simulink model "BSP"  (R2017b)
settings: Solver=FixedStepDiscrete  StartTime=0.0  StopTime=10.0  FixedStep=0.01  RelTol=1e-3  EnableMultiTasking=on
undefined symbols (not defined in the file): ASWTYPE_FALSE, ASWTYPE_TRUE, CcBSP_CellVoltRngHiThrd_mV, CcBSP_CellVoltRngLowThrd_mV, CcBSP_ChrgMaxCellTempSaf_C, CcBSP_DCChrgNegTempHiThrd_C, CcBSP_DCChrgPosTempHiThrd_C, CcBSP_MaxCellTempSaf_C, CcBSP_MaxCellVoltSafDiff_mV, CcBSP_MinCellVoltSafDiff_mV, CcBSP_PackCurrSaf_A, Enum_CTCCtrCtlConnMode, Enum_LDPCC2St, Enum_ODPCCState
libraries: AIWAYS_Powertrain_BMS_lib x14

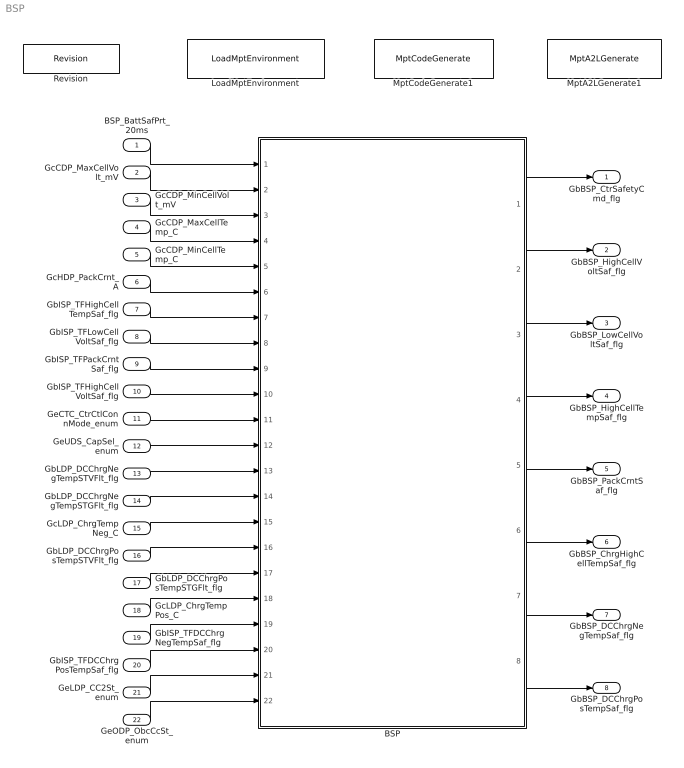
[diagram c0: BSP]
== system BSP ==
  BSP_BattSafPrt_20ms : Inport
  GcCDP_MaxCellVolt_mV : Inport  Port=2
  GcCDP_MinCellVolt_mV : Inport  Port=3
  GcCDP_MaxCellTemp_C : Inport  Port=4
  GcCDP_MinCellTemp_C : Inport  Port=5
  GcHDP_PackCrnt_A : Inport  Port=6
  GbISP_TFHighCellTempSaf_flg : Inport  Port=7
  GbISP_TFLowCellVoltSaf_flg : Inport  Port=8
  GbISP_TFPackCrntSaf_flg : Inport  Port=9
  GbISP_TFHighCellVoltSaf_flg : Inport  Port=10
  GeCTC_CtrCtlConnMode_enum : Inport  Port=11
  GeUDS_CapSel_enum : Inport  Port=12
  GbLDP_DCChrgNegTempSTVFlt_flg : Inport  Port=13
  GbLDP_DCChrgNegTempSTGFlt_flg : Inport  Port=14
  GcLDP_ChrgTempNeg_C : Inport  Port=15
  GbLDP_DCChrgPosTempSTVFlt_flg : Inport  Port=16
  GbLDP_DCChrgPosTempSTGFlt_flg : Inport  Port=17
  GcLDP_ChrgTempPos_C : Inport  Port=18
  GbISP_TFDCChrgNegTempSaf_flg : Inport  Port=19
  GbISP_TFDCChrgPosTempSaf_flg : Inport  Port=20
  GeLDP_CC2St_enum : Inport  Port=21
  GeODP_ObcCcSt_enum : Inport  Port=22
  BSP : Subsystem
  LoadMptEnvironment : AIWAYS_Powertrain_BMS_lib/Config/LoadMptEnvironment  ProjectName=Comm  SuppierID=NewPlatformUAES
  MptA2LGenerate1 : AIWAYS_Powertrain_BMS_lib/Config/MptA2LGenerate  SystemSampleTime=-1
  MptCodeGenerate1 : AIWAYS_Powertrain_BMS_lib/Config/MptCodeGenerate  SystemSampleTime=-1
  Revision : AIWAYS_Powertrain_BMS_lib/Config/Revision  curVersion='M105C111'  newVersion='M105C111'
  GbBSP_CtrSafetyCmd_flg : Outport
  GbBSP_HighCellVoltSaf_flg : Outport  Port=2
  GbBSP_LowCellVoltSaf_flg : Outport  Port=3
  GbBSP_HighCellTempSaf_flg : Outport  Port=4
  GbBSP_PackCrntSaf_flg : Outport  Port=5
  GbBSP_ChrgHighCellTempSaf_flg : Outport  Port=6
  GbBSP_DCChrgNegTempSaf_flg : Outport  Port=7
  GbBSP_DCChrgPosTempSaf_flg : Outport  Port=8
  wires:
  GcCDP_MaxCellVolt_mV/1 -> BSP/2(GcCDP_MaxCellVolt_mV)
  GcCDP_MinCellVolt_mV/1 -> BSP/3(GcCDP_MinCellVolt_mV)
  GcCDP_MaxCellTemp_C/1 -> BSP/4(GcCDP_MaxCellTemp_C)
  GcCDP_MinCellTemp_C/1 -> BSP/5(GcCDP_MinCellTemp_C)
  GcHDP_PackCrnt_A/1 -> BSP/6(GcHDP_PackCrnt_A)
  BSP_BattSafPrt_20ms/1 -> BSP/1(BSP_BattSafPrt_20ms)
  BSP/1(GbBSP_CtrSafetyCmd_flg) -> GbBSP_CtrSafetyCmd_flg/1
  BSP/2(GbBSP_HighCellVoltSaf_flg) -> GbBSP_HighCellVoltSaf_flg/1
  BSP/3(GbBSP_LowCellVoltSaf_flg) -> GbBSP_LowCellVoltSaf_flg/1
  BSP/4(GbBSP_HighCellTempSaf_flg) -> GbBSP_HighCellTempSaf_flg/1
  BSP/5(GbBSP_PackCrntSaf_flg) -> GbBSP_PackCrntSaf_flg/1
  GbISP_TFHighCellTempSaf_flg/1 -> BSP/7(GbISP_TFHighCellTempSaf_flg)
  GbISP_TFLowCellVoltSaf_flg/1 -> BSP/8(GbISP_TFLowCellVoltSaf_flg)
  GbISP_TFPackCrntSaf_flg/1 -> BSP/9(GbISP_TFPackCrntSaf_flg)
  GbISP_TFHighCellVoltSaf_flg/1 -> BSP/10(GbISP_TFHighCellVoltSaf_flg)
  BSP/6(GbBSP_ChrgHighCellTempSaf_flg) -> GbBSP_ChrgHighCellTempSaf_flg/1
  GeCTC_CtrCtlConnMode_enum/1 -> BSP/11(GeCTC_CtrCtlConnMode_enum)
  GeUDS_CapSel_enum/1 -> BSP/12(GeUDS_CapSel_enum)
  GbLDP_DCChrgNegTempSTVFlt_flg/1 -> BSP/13(GbLDP_DCChrgNegTempSTVFlt_flg)
  GbLDP_DCChrgNegTempSTGFlt_flg/1 -> BSP/14(GbLDP_DCChrgNegTempSTGFlt_flg)
  GcLDP_ChrgTempNeg_C/1 -> BSP/15(GcLDP_ChrgTempNeg_C)
  GbLDP_DCChrgPosTempSTVFlt_flg/1 -> BSP/16(GbLDP_DCChrgPosTempSTVFlt_flg)
  GbLDP_DCChrgPosTempSTGFlt_flg/1 -> BSP/17(GbLDP_DCChrgPosTempSTGFlt_flg)
  GcLDP_ChrgTempPos_C/1 -> BSP/18(GcLDP_ChrgTempPos_C)
  GbISP_TFDCChrgNegTempSaf_flg/1 -> BSP/19(GbISP_TFDCChrgNegTempSaf_flg)
  GbISP_TFDCChrgPosTempSaf_flg/1 -> BSP/20(GbISP_TFDCChrgPosTempSaf_flg)
  BSP/7(GbBSP_DCChrgNegTempSaf_flg) -> GbBSP_DCChrgNegTempSaf_flg/1
  BSP/8(GbBSP_DCChrgPosTempSaf_flg) -> GbBSP_DCChrgPosTempSaf_flg/1
  GeLDP_CC2St_enum/1 -> BSP/21(GeLDP_CC2St_enum)
  GeODP_ObcCcSt_enum/1 -> BSP/22(GeODP_ObcCcSt_enum)

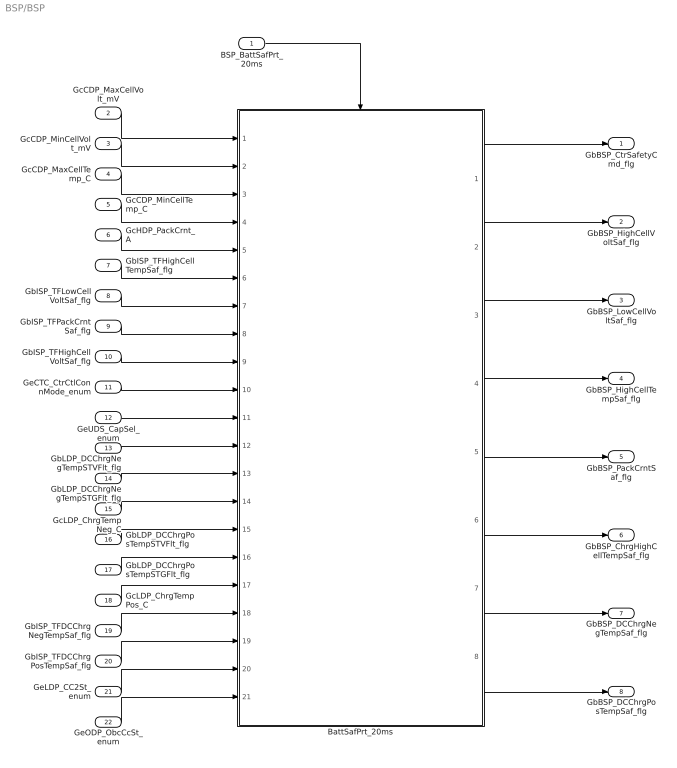
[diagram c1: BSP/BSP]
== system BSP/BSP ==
  BSP_BattSafPrt_20ms : Inport
  GcCDP_MaxCellVolt_mV : Inport  Port=2
  GcCDP_MinCellVolt_mV : Inport  Port=3
  GcCDP_MaxCellTemp_C : Inport  Port=4
  GcCDP_MinCellTemp_C : Inport  Port=5
  GcHDP_PackCrnt_A : Inport  Port=6
  GbISP_TFHighCellTempSaf_flg : Inport  Port=7
  GbISP_TFLowCellVoltSaf_flg : Inport  Port=8
  GbISP_TFPackCrntSaf_flg : Inport  Port=9
  GbISP_TFHighCellVoltSaf_flg : Inport  Port=10
  GeCTC_CtrCtlConnMode_enum : Inport  Port=11
  GeUDS_CapSel_enum : Inport  Port=12
  GbLDP_DCChrgNegTempSTVFlt_flg : Inport  Port=13
  GbLDP_DCChrgNegTempSTGFlt_flg : Inport  Port=14
  GcLDP_ChrgTempNeg_C : Inport  Port=15
  GbLDP_DCChrgPosTempSTVFlt_flg : Inport  Port=16
  GbLDP_DCChrgPosTempSTGFlt_flg : Inport  Port=17
  GcLDP_ChrgTempPos_C : Inport  Port=18
  GbISP_TFDCChrgNegTempSaf_flg : Inport  Port=19
  GbISP_TFDCChrgPosTempSaf_flg : Inport  Port=20
  GeLDP_CC2St_enum : Inport  Port=21
  GeODP_ObcCcSt_enum : Inport  Port=22
  BattSafPrt_20ms : Subsystem
  GbBSP_CtrSafetyCmd_flg : Outport
  GbBSP_HighCellVoltSaf_flg : Outport  Port=2
  GbBSP_LowCellVoltSaf_flg : Outport  Port=3
  GbBSP_HighCellTempSaf_flg : Outport  Port=4
  GbBSP_PackCrntSaf_flg : Outport  Port=5
  GbBSP_ChrgHighCellTempSaf_flg : Outport  Port=6
  GbBSP_DCChrgNegTempSaf_flg : Outport  Port=7
  GbBSP_DCChrgPosTempSaf_flg : Outport  Port=8
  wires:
  BSP_BattSafPrt_20ms/1 -> BattSafPrt_20ms/Trigger
  GcCDP_MaxCellVolt_mV/1 -> BattSafPrt_20ms/1(GcCDP_MaxCellVolt_mV)
  GcCDP_MinCellVolt_mV/1 -> BattSafPrt_20ms/2(GcCDP_MinCellVolt_mV)
  GcCDP_MaxCellTemp_C/1 -> BattSafPrt_20ms/3(GcCDP_MaxCellTemp_C)
  GcCDP_MinCellTemp_C/1 -> BattSafPrt_20ms/4(GcCDP_MinCellTemp_C)
  GcHDP_PackCrnt_A/1 -> BattSafPrt_20ms/5(GcHDP_PackCrnt_A)
  BattSafPrt_20ms/1(GbBSP_CtrSafetyCmd_flg) -> GbBSP_CtrSafetyCmd_flg/1
  BattSafPrt_20ms/2(GbBSP_HighCellVoltSaf_flg) -> GbBSP_HighCellVoltSaf_flg/1
  BattSafPrt_20ms/3(GbBSP_LowCellVoltSaf_flg) -> GbBSP_LowCellVoltSaf_flg/1
  BattSafPrt_20ms/4(GbBSP_HighCellTempSaf_flg) -> GbBSP_HighCellTempSaf_flg/1
  BattSafPrt_20ms/5(GbBSP_PackCrntSaf_flg) -> GbBSP_PackCrntSaf_flg/1
  GbISP_TFHighCellTempSaf_flg/1 -> BattSafPrt_20ms/6(GbISP_TFHighCellTempSaf_flg)
  GbISP_TFLowCellVoltSaf_flg/1 -> BattSafPrt_20ms/7(GbISP_TFLowCellVoltSaf_flg)
  GbISP_TFPackCrntSaf_flg/1 -> BattSafPrt_20ms/8(GbISP_TFPackCrntSaf_flg)
  GbISP_TFHighCellVoltSaf_flg/1 -> BattSafPrt_20ms/9(GbISP_TFHighCellVoltSaf_flg)
  GeCTC_CtrCtlConnMode_enum/1 -> BattSafPrt_20ms/10(GeCTC_CtrCtlConnMode_enum)
  BattSafPrt_20ms/6(GbBSP_ChrgHighCellTempSaf_flg) -> GbBSP_ChrgHighCellTempSaf_flg/1
  GeUDS_CapSel_enum/1 -> BattSafPrt_20ms/11(GeUDS_CapSel_enum)
  GbLDP_DCChrgNegTempSTVFlt_flg/1 -> BattSafPrt_20ms/12(GbLDP_DCChrgNegTempSTVFlt_flg)
  GbLDP_DCChrgNegTempSTGFlt_flg/1 -> BattSafPrt_20ms/13(GbLDP_DCChrgNegTempSTGFlt_flg)
  GcLDP_ChrgTempNeg_C/1 -> BattSafPrt_20ms/14(GcLDP_ChrgTempNeg_C)
  GbLDP_DCChrgPosTempSTVFlt_flg/1 -> BattSafPrt_20ms/15(GbLDP_DCChrgPosTempSTVFlt_flg)
  GbLDP_DCChrgPosTempSTGFlt_flg/1 -> BattSafPrt_20ms/16(GbLDP_DCChrgPosTempSTGFlt_flg)
  GcLDP_ChrgTempPos_C/1 -> BattSafPrt_20ms/17(GcLDP_ChrgTempPos_C)
  GbISP_TFDCChrgNegTempSaf_flg/1 -> BattSafPrt_20ms/18(GbISP_TFDCChrgNegTempSaf_flg)
  GbISP_TFDCChrgPosTempSaf_flg/1 -> BattSafPrt_20ms/19(GbISP_TFDCChrgPosTempSaf_flg)
  BattSafPrt_20ms/7(GbBSP_DCChrgNegTempSaf_flg) -> GbBSP_DCChrgNegTempSaf_flg/1
  BattSafPrt_20ms/8(GbBSP_DCChrgPosTempSaf_flg) -> GbBSP_DCChrgPosTempSaf_flg/1
  GeLDP_CC2St_enum/1 -> BattSafPrt_20ms/20(GeLDP_CC2St_enum)
  GeODP_ObcCcSt_enum/1 -> BattSafPrt_20ms/21(GeODP_ObcCcSt_enum)

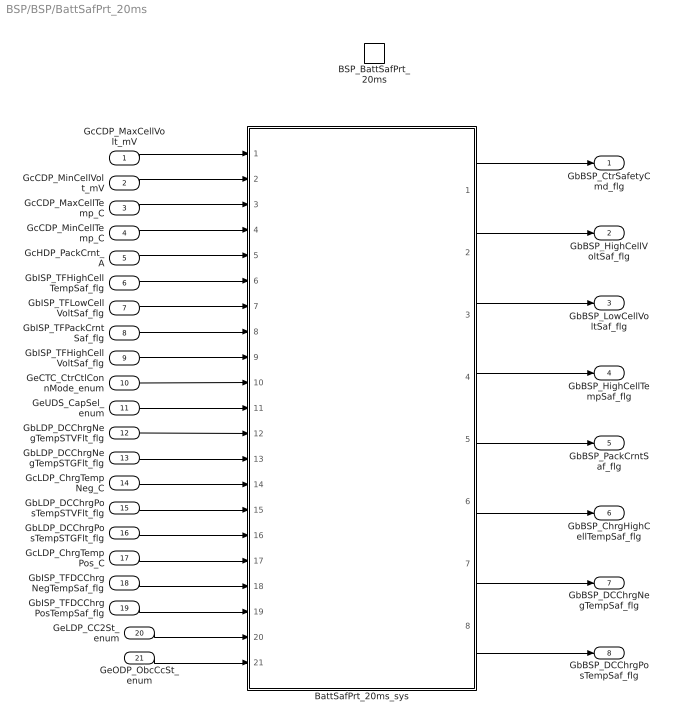
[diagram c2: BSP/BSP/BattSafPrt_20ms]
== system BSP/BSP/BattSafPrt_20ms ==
  GcCDP_MaxCellVolt_mV : Inport
  GcCDP_MinCellVolt_mV : Inport  Port=2
  GcCDP_MaxCellTemp_C : Inport  Port=3
  GcCDP_MinCellTemp_C : Inport  Port=4
  GcHDP_PackCrnt_A : Inport  Port=5
  GbISP_TFHighCellTempSaf_flg : Inport  Port=6
  GbISP_TFLowCellVoltSaf_flg : Inport  Port=7
  GbISP_TFPackCrntSaf_flg : Inport  Port=8
  GbISP_TFHighCellVoltSaf_flg : Inport  Port=9
  GeCTC_CtrCtlConnMode_enum : Inport  Port=10
  GeUDS_CapSel_enum : Inport  Port=11
  GbLDP_DCChrgNegTempSTVFlt_flg : Inport  Port=12
  GbLDP_DCChrgNegTempSTGFlt_flg : Inport  Port=13
  GcLDP_ChrgTempNeg_C : Inport  Port=14
  GbLDP_DCChrgPosTempSTVFlt_flg : Inport  Port=15
  GbLDP_DCChrgPosTempSTGFlt_flg : Inport  Port=16
  GcLDP_ChrgTempPos_C : Inport  Port=17
  GbISP_TFDCChrgNegTempSaf_flg : Inport  Port=18
  GbISP_TFDCChrgPosTempSaf_flg : Inport  Port=19
  GeLDP_CC2St_enum : Inport  Port=20
  GeODP_ObcCcSt_enum : Inport  Port=21
  BSP_BattSafPrt_20ms : TriggerPort  TriggerType=function-call  VariantControl=(inherit)
  BattSafPrt_20ms_sys : Subsystem
  GbBSP_CtrSafetyCmd_flg : Outport
  GbBSP_HighCellVoltSaf_flg : Outport  Port=2
  GbBSP_LowCellVoltSaf_flg : Outport  Port=3
  GbBSP_HighCellTempSaf_flg : Outport  Port=4
  GbBSP_PackCrntSaf_flg : Outport  Port=5
  GbBSP_ChrgHighCellTempSaf_flg : Outport  Port=6
  GbBSP_DCChrgNegTempSaf_flg : Outport  Port=7
  GbBSP_DCChrgPosTempSaf_flg : Outport  Port=8
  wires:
  GcCDP_MaxCellVolt_mV/1 -> BattSafPrt_20ms_sys/1(GcCDP_MaxCellVolt_mV)
  GcCDP_MinCellVolt_mV/1 -> BattSafPrt_20ms_sys/2(GcCDP_MinCellVolt_mV)
  GcCDP_MaxCellTemp_C/1 -> BattSafPrt_20ms_sys/3(GcCDP_MaxCellTemp_C)
  GcCDP_MinCellTemp_C/1 -> BattSafPrt_20ms_sys/4(GcCDP_MinCellTemp_C)
  GcHDP_PackCrnt_A/1 -> BattSafPrt_20ms_sys/5(GcHDP_PackCrnt_A)
  BattSafPrt_20ms_sys/1(GbBSP_CtrSafetyCmd_flg) -> GbBSP_CtrSafetyCmd_flg/1
  BattSafPrt_20ms_sys/2(GbBSP_HighCellVoltSaf_flg) -> GbBSP_HighCellVoltSaf_flg/1
  BattSafPrt_20ms_sys/3(GbBSP_LowCellVoltSaf_flg) -> GbBSP_LowCellVoltSaf_flg/1
  BattSafPrt_20ms_sys/4(GbBSP_HighCellTempSaf_flg) -> GbBSP_HighCellTempSaf_flg/1
  BattSafPrt_20ms_sys/5(GbBSP_PackCrntSaf_flg) -> GbBSP_PackCrntSaf_flg/1
  GbISP_TFHighCellTempSaf_flg/1 -> BattSafPrt_20ms_sys/6(GbISP_TFHighCellTempSaf_flg)
  GbISP_TFLowCellVoltSaf_flg/1 -> BattSafPrt_20ms_sys/7(GbISP_TFLowCellVoltSaf_flg)
  GbISP_TFPackCrntSaf_flg/1 -> BattSafPrt_20ms_sys/8(GbISP_TFPackCrntSaf_flg)
  GbISP_TFHighCellVoltSaf_flg/1 -> BattSafPrt_20ms_sys/9(GbISP_TFHighCellVoltSaf_flg)
  BattSafPrt_20ms_sys/6(GbBSP_ChrgHighCellTempSaf_flg) -> GbBSP_ChrgHighCellTempSaf_flg/1
  GeCTC_CtrCtlConnMode_enum/1 -> BattSafPrt_20ms_sys/10(GeCTC_CtrCtlConnMode_enum)
  GeUDS_CapSel_enum/1 -> BattSafPrt_20ms_sys/11(GeUDS_CapSel_enum)
  GbLDP_DCChrgNegTempSTVFlt_flg/1 -> BattSafPrt_20ms_sys/12(GbLDP_DCChrgNegTempSTVFlt_flg)
  GbLDP_DCChrgNegTempSTGFlt_flg/1 -> BattSafPrt_20ms_sys/13(GbLDP_DCChrgNegTempSTGFlt_flg)
  GcLDP_ChrgTempNeg_C/1 -> BattSafPrt_20ms_sys/14(GcLDP_ChrgTempNeg_C)
  GbLDP_DCChrgPosTempSTVFlt_flg/1 -> BattSafPrt_20ms_sys/15(GbLDP_DCChrgPosTempSTVFlt_flg)
  GbLDP_DCChrgPosTempSTGFlt_flg/1 -> BattSafPrt_20ms_sys/16(GbLDP_DCChrgPosTempSTGFlt_flg)
  GcLDP_ChrgTempPos_C/1 -> BattSafPrt_20ms_sys/17(GcLDP_ChrgTempPos_C)
  GbISP_TFDCChrgNegTempSaf_flg/1 -> BattSafPrt_20ms_sys/18(GbISP_TFDCChrgNegTempSaf_flg)
  GbISP_TFDCChrgPosTempSaf_flg/1 -> BattSafPrt_20ms_sys/19(GbISP_TFDCChrgPosTempSaf_flg)
  BattSafPrt_20ms_sys/8(GbBSP_DCChrgPosTempSaf_flg) -> GbBSP_DCChrgPosTempSaf_flg/1
  BattSafPrt_20ms_sys/7(GbBSP_DCChrgNegTempSaf_flg) -> GbBSP_DCChrgNegTempSaf_flg/1
  GeLDP_CC2St_enum/1 -> BattSafPrt_20ms_sys/20(GeLDP_CC2St_enum)
  GeODP_ObcCcSt_enum/1 -> BattSafPrt_20ms_sys/21(GeODP_ObcCcSt_enum)

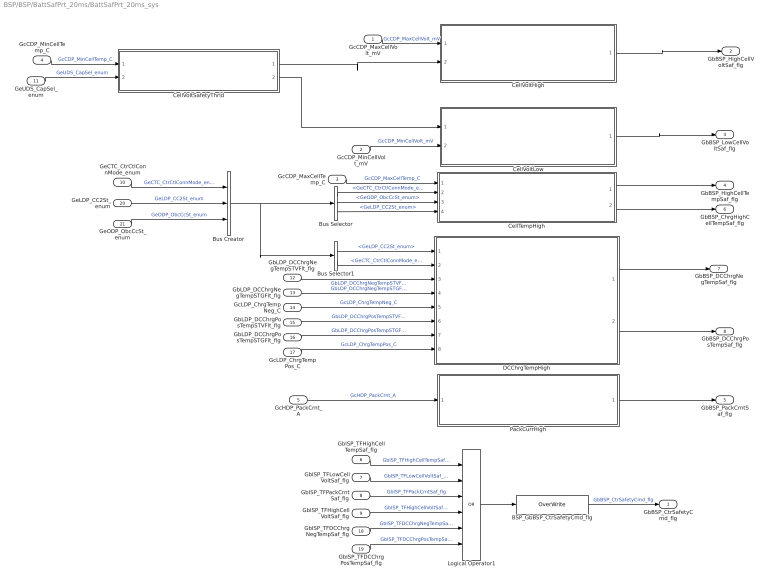
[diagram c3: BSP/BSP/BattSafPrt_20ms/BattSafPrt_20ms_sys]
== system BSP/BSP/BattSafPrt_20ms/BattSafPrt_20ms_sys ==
  GcCDP_MaxCellVolt_mV : Inport
  GcCDP_MinCellVolt_mV : Inport  Port=2
  GcCDP_MaxCellTemp_C : Inport  Port=3
  GcCDP_MinCellTemp_C : Inport  Port=4
  GcHDP_PackCrnt_A : Inport  Port=5
  GbISP_TFHighCellTempSaf_flg : Inport  Port=6
  GbISP_TFLowCellVoltSaf_flg : Inport  Port=7
  GbISP_TFPackCrntSaf_flg : Inport  Port=8
  GbISP_TFHighCellVoltSaf_flg : Inport  Port=9
  GeCTC_CtrCtlConnMode_enum : Inport  Port=10
  GeUDS_CapSel_enum : Inport  Port=11
  GbLDP_DCChrgNegTempSTVFlt_flg : Inport  Port=12
  GbLDP_DCChrgNegTempSTGFlt_flg : Inport  Port=13
  GcLDP_ChrgTempNeg_C : Inport  Port=14
  GbLDP_DCChrgPosTempSTVFlt_flg : Inport  Port=15
  GbLDP_DCChrgPosTempSTGFlt_flg : Inport  Port=16
  GcLDP_ChrgTempPos_C : Inport  Port=17
  GbISP_TFDCChrgNegTempSaf_flg : Inport  Port=18
  GbISP_TFDCChrgPosTempSaf_flg : Inport  Port=19
  GeLDP_CC2St_enum : Inport  Port=20
  GeODP_ObcCcSt_enum : Inport  Port=21
  BSP_GbBSP_CtrSafetyCmd_flg : AIWAYS_Powertrain_BMS_lib/Signals/OverWrite  OverWrite_Value=CbBSP_CtrSafetyCmdOvr_flg  OverWrite_flag=CbBSP_CtrSafetyCmdOvrSwt_flg
  Bus Creator : BusCreator  Inputs=3
  Bus Selector : BusSelector  OutputSignals=GeCTC_CtrCtlConnMode_enum,GeODP_ObcCcSt_enum,GeLDP_CC2St_enum
  Bus Selector1 : BusSelector  OutputSignals=GeLDP_CC2St_enum,GeCTC_CtrCtlConnMode_enum
  CellTempHigh : Subsystem
  CellVoltHigh : Subsystem
  CellVoltLow : Subsystem
  CellVoltSafetyThrld : Subsystem
  DCChrgTempHigh : Subsystem
  Logical Operator1 : Logic  Operator=OR  Inputs=6  AllPortsSameDT=off  OutDataTypeStr=boolean
  PackCurrHigh : Subsystem
  GbBSP_CtrSafetyCmd_flg : Outport
  GbBSP_HighCellVoltSaf_flg : Outport  Port=2
  GbBSP_LowCellVoltSaf_flg : Outport  Port=3
  GbBSP_HighCellTempSaf_flg : Outport  Port=4
  GbBSP_PackCrntSaf_flg : Outport  Port=5
  GbBSP_ChrgHighCellTempSaf_flg : Outport  Port=6
  GbBSP_DCChrgNegTempSaf_flg : Outport  Port=7
  GbBSP_DCChrgPosTempSaf_flg : Outport  Port=8
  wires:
  GcCDP_MinCellTemp_C/1 -> CellVoltSafetyThrld/1(GcCDP_MinCellTemp_C)  "GcCDP_MinCellTemp_C"
  GcCDP_MaxCellVolt_mV/1 -> CellVoltHigh/1(GcCDP_MaxCellVolt_mV)  "GcCDP_MaxCellVolt_mV"
  CellVoltSafetyThrld/1(LcBSP_MaxCellVoltSafetyThrld_mV) -> CellVoltHigh/2(LcBSP_MaxCellVoltSafetyThrld_mV)
  CellVoltSafetyThrld/2(LcBSP_MinCellVoltSafetyThrld_mV) -> CellVoltLow/1(LcBSP_MinCellVoltSafetyThrld_mV)
  GcCDP_MinCellVolt_mV/1 -> CellVoltLow/2(GcCDP_MinCellVolt_mV)  "GcCDP_MinCellVolt_mV"
  GcCDP_MaxCellTemp_C/1 -> CellTempHigh/1(GcCDP_MaxCellTemp_C)  "GcCDP_MaxCellTemp_C"
  GcHDP_PackCrnt_A/1 -> PackCurrHigh/1(GcHDP_PackCrnt_A)  "GcHDP_PackCrnt_A"
  CellVoltHigh/1(GbBSP_HighCellVoltSaf_flg) -> GbBSP_HighCellVoltSaf_flg/1
  CellVoltLow/1(GbBSP_LowCellVoltSaf_flg) -> GbBSP_LowCellVoltSaf_flg/1
  CellTempHigh/1(GbBSP_HighCellTempSaf_flg) -> GbBSP_HighCellTempSaf_flg/1
  PackCurrHigh/1(GbBSP_PackCrntSaf_flg) -> GbBSP_PackCrntSaf_flg/1
  Logical Operator1/1 -> BSP_GbBSP_CtrSafetyCmd_flg/1
  BSP_GbBSP_CtrSafetyCmd_flg/1 -> GbBSP_CtrSafetyCmd_flg/1  "GbBSP_CtrSafetyCmd_flg"
  GbISP_TFHighCellTempSaf_flg/1 -> Logical Operator1/1  "GbISP_TFHighCellTempSaf_flg"
  GbISP_TFLowCellVoltSaf_flg/1 -> Logical Operator1/2  "GbISP_TFLowCellVoltSaf_flg"
  GbISP_TFPackCrntSaf_flg/1 -> Logical Operator1/3  "GbISP_TFPackCrntSaf_flg"
  GbISP_TFHighCellVoltSaf_flg/1 -> Logical Operator1/4  "GbISP_TFHighCellVoltSaf_flg"
  CellTempHigh/2(GbBSP_ChrgHighCellTempSaf_flg) -> GbBSP_ChrgHighCellTempSaf_flg/1
  GeUDS_CapSel_enum/1 -> CellVoltSafetyThrld/2(GeUDS_CapSel_enum)  "GeUDS_CapSel_enum"
  GbLDP_DCChrgNegTempSTVFlt_flg/1 -> DCChrgTempHigh/3(GbLDP_DCChrgNegTempSTVFlt_flg)  "GbLDP_DCChrgNegTempSTVFlt_flg"
  GbLDP_DCChrgNegTempSTGFlt_flg/1 -> DCChrgTempHigh/4(GbLDP_DCChrgNegTempSTGFlt_flg)  "GbLDP_DCChrgNegTempSTGFlt_flg"
  GcLDP_ChrgTempNeg_C/1 -> DCChrgTempHigh/5(GcLDP_ChrgTempNeg_C)  "GcLDP_ChrgTempNeg_C"
  GbLDP_DCChrgPosTempSTVFlt_flg/1 -> DCChrgTempHigh/6(GbLDP_DCChrgPosTempSTVFlt_flg)  "GbLDP_DCChrgPosTempSTVFlt_flg"
  GbLDP_DCChrgPosTempSTGFlt_flg/1 -> DCChrgTempHigh/7(GbLDP_DCChrgPosTempSTGFlt_flg)  "GbLDP_DCChrgPosTempSTGFlt_flg"
  GcLDP_ChrgTempPos_C/1 -> DCChrgTempHigh/8(GcLDP_ChrgTempPos_C)  "GcLDP_ChrgTempPos_C"
  DCChrgTempHigh/2(GbBSP_DCChrgPosTempSaf_flg) -> GbBSP_DCChrgPosTempSaf_flg/1
  DCChrgTempHigh/1(GbBSP_DCChrgNegTempSaf_flg) -> GbBSP_DCChrgNegTempSaf_flg/1
  GbISP_TFDCChrgNegTempSaf_flg/1 -> Logical Operator1/5  "GbISP_TFDCChrgNegTempSaf_flg"
  GbISP_TFDCChrgPosTempSaf_flg/1 -> Logical Operator1/6  "GbISP_TFDCChrgPosTempSaf_flg"
  GeLDP_CC2St_enum/1 -> Bus Creator/2  "GeLDP_CC2St_enum"
  GeCTC_CtrCtlConnMode_enum/1 -> Bus Creator/1  "GeCTC_CtrCtlConnMode_enum"
  GeODP_ObcCcSt_enum/1 -> Bus Creator/3  "GeODP_ObcCcSt_enum"
  Bus Creator/1 -> Bus Selector1/1, Bus Selector/1
  Bus Selector/1 -> CellTempHigh/2(GeCTC_CtrCtlConnMode_enum)  "<GeCTC_CtrCtlConnMode_enum>"
  Bus Selector/2 -> CellTempHigh/3(GeODP_ObcCcSt_enum)  "<GeODP_ObcCcSt_enum>"
  Bus Selector/3 -> CellTempHigh/4(GeLDP_CC2St_enum)  "<GeLDP_CC2St_enum>"
  Bus Selector1/1 -> DCChrgTempHigh/1(GeLDP_CC2St_enum)  "<GeLDP_CC2St_enum>"
  Bus Selector1/2 -> DCChrgTempHigh/2(GeCTC_CtrCtlConnMode_enum)  "<GeCTC_CtrCtlConnMode_enum>"

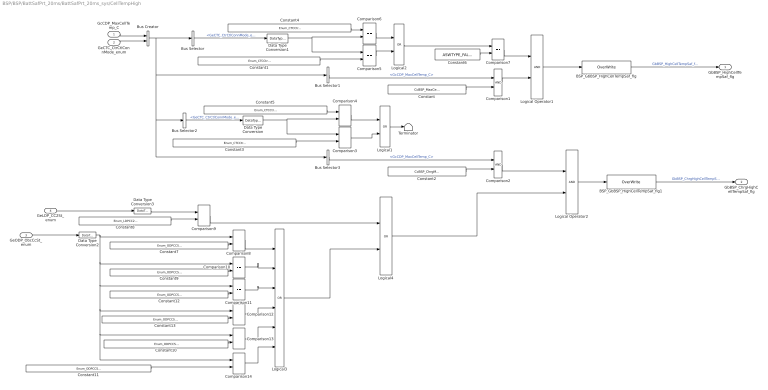
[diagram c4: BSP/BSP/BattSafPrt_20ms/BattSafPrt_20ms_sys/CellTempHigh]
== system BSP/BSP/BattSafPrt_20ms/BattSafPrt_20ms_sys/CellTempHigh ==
  GcCDP_MaxCellTemp_C : Inport
  GeCTC_CtrCtlConnMode_enum : Inport  Port=2
  GeODP_ObcCcSt_enum : Inport  Port=3
  GeLDP_CC2St_enum : Inport  Port=4
  BSP_GbBSP_HighCellTempSaf_flg : AIWAYS_Powertrain_BMS_lib/Signals/OverWrite  OverWrite_Value=CbBSP_HighCellTempSafOvr_flg  OverWrite_flag=CbBSP_HighCellTempSafOvrSwt_flg
  BSP_GbBSP_HighCellTempSaf_flg1 : AIWAYS_Powertrain_BMS_lib/Signals/OverWrite  OverWrite_Value=CbBSP_ChrgHighCellTempSafOvr_flg  OverWrite_flag=CbBSP_ChrgHighCellTempSafOvrSwt_flg
  Bus Creator : BusCreator  Inputs=2
  Bus Selector : BusSelector  OutputSignals=GeCTC_CtrCtlConnMode_enum
  Bus Selector1 : BusSelector  OutputSignals=GcCDP_MaxCellTemp_C
  Bus Selector2 : BusSelector  OutputSignals=GeCTC_CtrCtlConnMode_enum
  Bus Selector3 : BusSelector  OutputSignals=GcCDP_MaxCellTemp_C
  Comparison1 : RelationalOperator  OutDataTypeStr=boolean
  Comparison{3..14} (12 alike) : RelationalOperator  Operator===  OutDataTypeStr=boolean
  Comparison2 : RelationalOperator  OutDataTypeStr=boolean
  Constant : Constant  Value=CcBSP_MaxCellTempSaf_C
  Constant1 : Constant  Value=Enum_CTCCtrCtlConnMode.Enum_CTCCtrCtlConnMode_ACChrg
  Constant10 : Constant  Value=Enum_ODPCCState.Enum_ODPCCState_DisChrgConnect16A2000
  Constant11 : Constant  Value=Enum_ODPCCState.Enum_ODPCCState_DisChrgConnect32A1000
  Constant12 : Constant  Value=Enum_ODPCCState.Enum_ODPCCState_ChrgConnect32A220
  Constant13 : Constant  Value=Enum_ODPCCState.Enum_ODPCCState_DisChrgConnect10A2700
  Constant2 : Constant  Value=CcBSP_ChrgMaxCellTempSaf_C
  Constant3 : Constant  Value=Enum_CTCCtrCtlConnMode.Enum_CTCCtrCtlConnMode_ACChrg
  Constant4 : Constant  Value=Enum_CTCCtrCtlConnMode.Enum_CTCCtrCtlConnMode_DCChrg
  Constant5 : Constant  Value=Enum_CTCCtrCtlConnMode.Enum_CTCCtrCtlConnMode_DCChrg
  Constant6 : Constant  Value=ASWTYPE_FALSE
  Constant7 : Constant  Value=Enum_ODPCCState.Enum_ODPCCState_ChrgConnect10A1500
  Constant8 : Constant  Value=Enum_LDPCC2St.Enum_LDPCC2St_Connect
  Constant9 : Constant  Value=Enum_ODPCCState.Enum_ODPCCState_ChrgConnect16A680
  Data Type Conversion{,1..3} (4 alike) : DataTypeConversion
  Logical Operator1 : Logic  AllPortsSameDT=off  OutDataTypeStr=boolean
  Logical Operator2 : Logic  AllPortsSameDT=off  OutDataTypeStr=boolean
  Logical1 : Logic  Operator=OR  OutDataTypeStr=boolean
  Logical2 : Logic  Operator=OR  OutDataTypeStr=boolean
  Logical3 : Logic  Operator=OR  Inputs=6  OutDataTypeStr=boolean
  Logical4 : Logic  Operator=OR  OutDataTypeStr=boolean
  Terminator : Terminator
  GbBSP_HighCellTempSaf_flg : Outport
  GbBSP_ChrgHighCellTempSaf_flg : Outport  Port=2
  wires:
  Constant/1 -> Comparison1/2
  BSP_GbBSP_HighCellTempSaf_flg/1 -> GbBSP_HighCellTempSaf_flg/1  "GbBSP_HighCellTempSaf_flg"
  Comparison1/1 -> Logical Operator1/2
  Logical Operator1/1 -> BSP_GbBSP_HighCellTempSaf_flg/1
  Bus Selector3/1 -> Comparison2/1  "<GcCDP_MaxCellTemp_C>"
  Constant2/1 -> Comparison2/2
  Comparison2/1 -> Logical Operator2/1
  Logical Operator2/1 -> BSP_GbBSP_HighCellTempSaf_flg1/1
  Logical1/1 -> Terminator/1
  Data Type Conversion/1 -> Comparison3/1, Comparison4/2
  BSP_GbBSP_HighCellTempSaf_flg1/1 -> GbBSP_ChrgHighCellTempSaf_flg/1  "GbBSP_ChrgHighCellTempSaf_flg"
  GeCTC_CtrCtlConnMode_enum/1 -> Bus Creator/2
  Constant3/1 -> Comparison3/2
  Comparison4/1 -> Logical1/1
  Constant5/1 -> Comparison4/1
  Comparison3/1 -> Logical1/2
  GcCDP_MaxCellTemp_C/1 -> Bus Creator/1
  Bus Creator/1 -> Bus Selector3/1, Bus Selector2/1, Bus Selector1/1, Bus Selector/1
  Comparison5/1 -> Logical2/2
  Constant4/1 -> Comparison6/1
  Comparison6/1 -> Logical2/1
  Constant1/1 -> Comparison5/2
  Data Type Conversion1/1 -> Comparison6/2, Comparison5/1
  Logical2/1 -> Comparison7/1
  Bus Selector/1 -> Data Type Conversion1/1  "<GeCTC_CtrCtlConnMode_enum>"
  Constant6/1 -> Comparison7/2
  Comparison7/1 -> Logical Operator1/1
  Bus Selector1/1 -> Comparison1/1  "<GcCDP_MaxCellTemp_C>"
  Bus Selector2/1 -> Data Type Conversion/1  "<GeCTC_CtrCtlConnMode_enum>"
  Constant10/1 -> Comparison13/2
  Comparison12/1 -> Logical3/4
  Constant7/1 -> Comparison8/2
  Data Type Conversion2/1 -> Comparison14/1, Comparison13/1, Comparison12/1, Comparison11/1, Comparison10/1, Comparison8/1
  Constant13/1 -> Comparison12/2
  Comparison13/1 -> Logical3/5
  Constant8/1 -> Comparison9/2
  Comparison14/1 -> Logical3/6
  GeLDP_CC2St_enum/1 -> Data Type Conversion3/1
  Constant12/1 -> Comparison11/2
  Constant11/1 -> Comparison14/2
  Comparison8/1 -> Logical3/1
  Constant9/1 -> Comparison10/2
  Logical3/1 -> Logical4/2
  Data Type Conversion3/1 -> Comparison9/1
  Comparison11/1 -> Logical3/3
  Comparison10/1 -> Logical3/2
  GeODP_ObcCcSt_enum/1 -> Data Type Conversion2/1
  Comparison9/1 -> Logical4/1
  Logical4/1 -> Logical Operator2/2

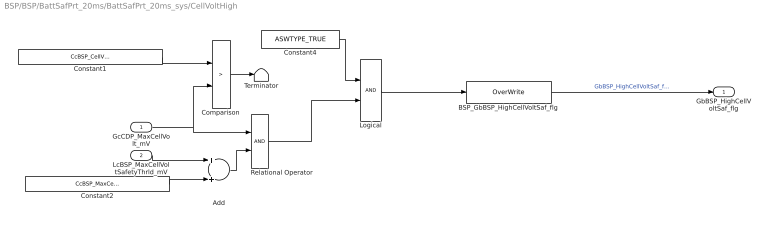
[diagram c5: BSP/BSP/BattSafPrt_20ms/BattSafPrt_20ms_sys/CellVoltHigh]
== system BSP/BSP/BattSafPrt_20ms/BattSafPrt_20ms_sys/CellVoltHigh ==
  GcCDP_MaxCellVolt_mV : Inport
  LcBSP_MaxCellVoltSafetyThrld_mV : Inport  Port=2
  Add : Sum
  BSP_GbBSP_HighCellVoltSaf_flg : AIWAYS_Powertrain_BMS_lib/Signals/OverWrite  OverWrite_Value=CbBSP_HighCellVoltSafOvr_flg  OverWrite_flag=CbBSP_HighCellVoltSafOvrSwt_flg
  Comparison : RelationalOperator  Operator=>  OutDataTypeStr=boolean
  Constant1 : Constant  Value=CcBSP_CellVoltRngHiThrd_mV
  Constant2 : Constant  Value=CcBSP_MaxCellVoltSafDiff_mV
  Constant4 : Constant  Value=ASWTYPE_TRUE
  Logical : Logic  OutDataTypeStr=boolean
  Relational Operator : RelationalOperator  OutDataTypeStr=boolean
  Terminator : Terminator
  GbBSP_HighCellVoltSaf_flg : Outport
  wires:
  GcCDP_MaxCellVolt_mV/1 -> Comparison/2, Relational Operator/1
  BSP_GbBSP_HighCellVoltSaf_flg/1 -> GbBSP_HighCellVoltSaf_flg/1  "GbBSP_HighCellVoltSaf_flg"
  Logical/1 -> BSP_GbBSP_HighCellVoltSaf_flg/1
  Add/1 -> Relational Operator/2
  LcBSP_MaxCellVoltSafetyThrld_mV/1 -> Add/1
  Constant2/1 -> Add/2
  Relational Operator/1 -> Logical/2
  Constant1/1 -> Comparison/1
  Comparison/1 -> Terminator/1
  Constant4/1 -> Logical/1

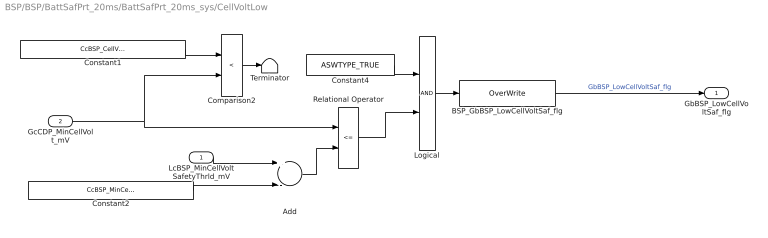
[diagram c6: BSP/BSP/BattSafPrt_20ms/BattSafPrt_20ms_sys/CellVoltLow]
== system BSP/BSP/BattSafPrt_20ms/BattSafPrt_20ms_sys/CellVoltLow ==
  LcBSP_MinCellVoltSafetyThrld_mV : Inport
  GcCDP_MinCellVolt_mV : Inport  Port=2
  Add : Sum  Inputs=+-
  BSP_GbBSP_LowCellVoltSaf_flg : AIWAYS_Powertrain_BMS_lib/Signals/OverWrite  OverWrite_Value=CbBSP_LowCellVoltSafOvr_flg  OverWrite_flag=CbBSP_LowCellVoltSafOvrSwt_flg
  Comparison2 : RelationalOperator  Operator=<  OutDataTypeStr=boolean
  Constant1 : Constant  Value=CcBSP_CellVoltRngLowThrd_mV
  Constant2 : Constant  Value=CcBSP_MinCellVoltSafDiff_mV
  Constant4 : Constant  Value=ASWTYPE_TRUE
  Logical : Logic  OutDataTypeStr=boolean
  Relational Operator : RelationalOperator  Operator=<=  OutDataTypeStr=boolean
  Terminator : Terminator
  GbBSP_LowCellVoltSaf_flg : Outport
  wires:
  GcCDP_MinCellVolt_mV/1 -> Relational Operator/1, Comparison2/2
  BSP_GbBSP_LowCellVoltSaf_flg/1 -> GbBSP_LowCellVoltSaf_flg/1  "GbBSP_LowCellVoltSaf_flg"
  Relational Operator/1 -> Logical/2
  Add/1 -> Relational Operator/2
  LcBSP_MinCellVoltSafetyThrld_mV/1 -> Add/1
  Constant2/1 -> Add/2
  Constant1/1 -> Comparison2/1
  Comparison2/1 -> Terminator/1
  Logical/1 -> BSP_GbBSP_LowCellVoltSaf_flg/1
  Constant4/1 -> Logical/1

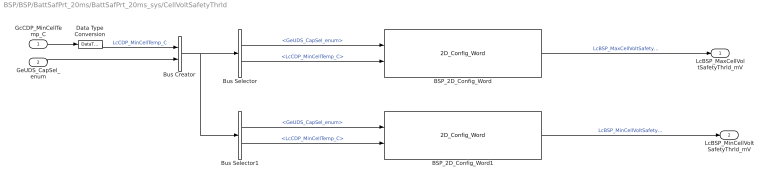
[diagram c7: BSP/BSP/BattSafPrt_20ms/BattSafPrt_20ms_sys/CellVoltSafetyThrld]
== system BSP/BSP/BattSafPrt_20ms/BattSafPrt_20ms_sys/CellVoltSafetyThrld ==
  GcCDP_MinCellTemp_C : Inport
  GeUDS_CapSel_enum : Inport  Port=2
  BSP_2D_Config_Word : AIWAYS_Powertrain_BMS_lib/Signals/2D_Config_Word  Default_Cal_Breakpoint1_Name=CaBSP_MaxCellVoltSafTempTab_C  Default_Cal_Table1_Name=CaBSP_CATL177MaxCellVoltSafVoltTab_mV  CATL153Ah_Cal_Breakpoint1_Name=CaBSP_MaxCellVoltSafTempTab_C  CATL153Ah_Cal_Table1_Name=CaBSP_CATL177MaxCellVoltSafVoltTab_mV  CATL180Ah_Cal_Breakpoint1_Name=CaBSP_MaxCellVoltSafTempTab_C  CATL180Ah_Cal_Table1_Name=CaBSP_CATL177MaxCellVoltSafVoltTab_mV  CATL177Ah_Cal_Breakpoint1_Name=CaBSP_MaxCellVoltSafTempTab_C  CATL177Ah_Cal_Table1_Name=CaBSP_CATL177MaxCellVoltSafVoltTab_mV  CATL203Ah_Cal_Breakpoint1_Name=CaBSP_MaxCellVoltSafTempTab_C  CATL203Ah_Cal_Table1_Name=CaBSP_CATL203MaxCellVoltSafVoltTab_mV  CATL51Ah_Cal_Breakpoint1_Name=CaBSP_MaxCellVoltSafTempTab_C  CATL51Ah_Cal_Table1_Name=CaBSP_CATL177MaxCellVoltSafVoltTab_mV  CATL132Ah_Cal_Breakpoint1_Name=CaBSP_MaxCellVoltSafTempTab_C  CATL132Ah_Cal_Table1_Name=CaBSP_CATL177MaxCellVoltSafVoltTab_mV  XWD75Ah_Cal_Breakpoint1_Name=CaBSP_MaxCellVoltSafTempTab_C  XWD75Ah_Cal_Table1_Name=CaBSP_XWD75MaxCellVoltSafVoltTab_mV  TFE177Ah_Cal_Breakpoint1_Name=CaBSP_MaxCellVoltSafTempTab_C  TFE177Ah_Cal_Table1_Name=CaBSP_TFE177MaxCellVoltSafVoltTab_mV  CATLCTP248Ah_Cal_Breakpoint1_Name=CaBSP_MaxCellVoltSafTempTab_C  CATLCTP248Ah_Cal_Table1_Name=CaBSP_CATL177MaxCellVoltSafVoltTab_mV
      link override Switch Case Action Subsystem8/1-D_Lookup_Table: BreakpointsForDimension1=CaBSP_MaxCellVoltSafTempTab_C  Table=CaBSP_TFE177MaxCellVoltSafVoltTab_mV
  BSP_2D_Config_Word1 : AIWAYS_Powertrain_BMS_lib/Signals/2D_Config_Word  Default_Cal_Breakpoint1_Name=CaBSP_MinCellVoltSafTempTab_C  Default_Cal_Table1_Name=CaBSP_CATL177MinCellVoltSafVoltTab_mV  CATL153Ah_Cal_Breakpoint1_Name=CaBSP_MinCellVoltSafTempTab_C  CATL153Ah_Cal_Table1_Name=CaBSP_CATL177MinCellVoltSafVoltTab_mV  CATL180Ah_Cal_Breakpoint1_Name=CaBSP_MinCellVoltSafTempTab_C  CATL180Ah_Cal_Table1_Name=CaBSP_CATL177MinCellVoltSafVoltTab_mV  CATL177Ah_Cal_Breakpoint1_Name=CaBSP_MinCellVoltSafTempTab_C  CATL177Ah_Cal_Table1_Name=CaBSP_CATL177MinCellVoltSafVoltTab_mV  CATL203Ah_Cal_Breakpoint1_Name=CaBSP_MinCellVoltSafTempTab_C  CATL203Ah_Cal_Table1_Name=CaBSP_CATL203MinCellVoltSafVoltTab_mV  CATL51Ah_Cal_Breakpoint1_Name=CaBSP_MinCellVoltSafTempTab_C  CATL51Ah_Cal_Table1_Name=CaBSP_CATL177MinCellVoltSafVoltTab_mV  CATL132Ah_Cal_Breakpoint1_Name=CaBSP_MinCellVoltSafTempTab_C  CATL132Ah_Cal_Table1_Name=CaBSP_CATL177MinCellVoltSafVoltTab_mV  XWD75Ah_Cal_Breakpoint1_Name=CaBSP_MinCellVoltSafTempTab_C  XWD75Ah_Cal_Table1_Name=CaBSP_XWD75MinCellVoltSafVoltTab_mV  TFE177Ah_Cal_Breakpoint1_Name=CaBSP_TFE177MinCellVoltSafTempTab_C  TFE177Ah_Cal_Table1_Name=CaBSP_TFE177MinCellVoltSafVoltTab_mV  CATLCTP248Ah_Cal_Breakpoint1_Name=CaBSP_MinCellVoltSafTempTab_C  CATLCTP248Ah_Cal_Table1_Name=CaBSP_CATL177MinCellVoltSafVoltTab_mV
      link override Switch Case Action Subsystem8/1-D_Lookup_Table: BreakpointsForDimension1=CaBSP_TFE177MinCellVoltSafTempTab_C  Table=CaBSP_TFE177MinCellVoltSafVoltTab_mV
  Bus Creator : BusCreator  Inputs=2
  Bus Selector : BusSelector  OutputSignals=GeUDS_CapSel_enum,LcCDP_MinCellTemp_C
  Bus Selector1 : BusSelector  OutputSignals=GeUDS_CapSel_enum,LcCDP_MinCellTemp_C
  Data Type Conversion : DataTypeConversion  OutDataTypeStr=fixdt(0,8,1,-40)
  LcBSP_MaxCellVoltSafetyThrld_mV : Outport
  LcBSP_MinCellVoltSafetyThrld_mV : Outport  Port=2
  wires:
  GcCDP_MinCellTemp_C/1 -> Data Type Conversion/1
  BSP_2D_Config_Word/1 -> LcBSP_MaxCellVoltSafetyThrld_mV/1  "LcBSP_MaxCellVoltSafetyThrld_mV"
  BSP_2D_Config_Word1/1 -> LcBSP_MinCellVoltSafetyThrld_mV/1  "LcBSP_MinCellVoltSafetyThrld_mV"
  Data Type Conversion/1 -> Bus Creator/1  "LcCDP_MinCellTemp_C"
  GeUDS_CapSel_enum/1 -> Bus Creator/2
  Bus Creator/1 -> Bus Selector1/1, Bus Selector/1
  Bus Selector/1 -> BSP_2D_Config_Word/1  "<GeUDS_CapSel_enum>"
  Bus Selector/2 -> BSP_2D_Config_Word/2  "<LcCDP_MinCellTemp_C>"
  Bus Selector1/1 -> BSP_2D_Config_Word1/1  "<GeUDS_CapSel_enum>"
  Bus Selector1/2 -> BSP_2D_Config_Word1/2  "<LcCDP_MinCellTemp_C>"

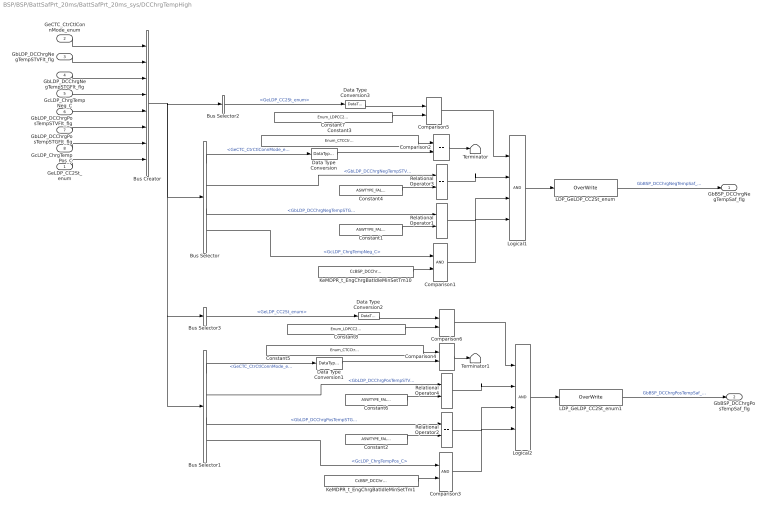
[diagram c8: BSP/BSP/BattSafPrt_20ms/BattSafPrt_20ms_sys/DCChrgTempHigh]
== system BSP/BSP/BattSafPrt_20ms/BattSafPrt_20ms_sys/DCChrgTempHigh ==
  GeLDP_CC2St_enum : Inport
  GeCTC_CtrCtlConnMode_enum : Inport  Port=2
  GbLDP_DCChrgNegTempSTVFlt_flg : Inport  Port=3
  GbLDP_DCChrgNegTempSTGFlt_flg : Inport  Port=4
  GcLDP_ChrgTempNeg_C : Inport  Port=5
  GbLDP_DCChrgPosTempSTVFlt_flg : Inport  Port=6
  GbLDP_DCChrgPosTempSTGFlt_flg : Inport  Port=7
  GcLDP_ChrgTempPos_C : Inport  Port=8
  Bus Creator : BusCreator  Inputs=8
  Bus Selector : BusSelector  OutputSignals=GeCTC_CtrCtlConnMode_enum,GbLDP_DCChrgNegTempSTVFlt_flg,GbLDP_DCChrgNegTempSTGFlt_flg,GcLDP_ChrgTempNeg_C
  Bus Selector1 : BusSelector  OutputSignals=GeCTC_CtrCtlConnMode_enum,GbLDP_DCChrgPosTempSTVFlt_flg,GbLDP_DCChrgPosTempSTGFlt_flg,GcLDP_ChrgTempPos_C
  Bus Selector2 : BusSelector  OutputSignals=GeLDP_CC2St_enum
  Bus Selector3 : BusSelector  OutputSignals=GeLDP_CC2St_enum
  Comparison1 : RelationalOperator  OutDataTypeStr=boolean
  Comparison{2,4..6} (4 alike) : RelationalOperator  Operator===  OutDataTypeStr=boolean
  Comparison3 : RelationalOperator  OutDataTypeStr=boolean
  Constant{1..2,4,6} (4 alike) : Constant  Value=ASWTYPE_FALSE
  Constant3 : Constant  Value=Enum_CTCCtrCtlConnMode.Enum_CTCCtrCtlConnMode_DCChrg
  Constant5 : Constant  Value=Enum_CTCCtrCtlConnMode.Enum_CTCCtrCtlConnMode_DCChrg
  Constant7 : Constant  Value=Enum_LDPCC2St.Enum_LDPCC2St_Connect
  Constant8 : Constant  Value=Enum_LDPCC2St.Enum_LDPCC2St_Connect
  Data Type Conversion{,1..3} (4 alike) : DataTypeConversion
  KeMDPR_t_EngChrgBatIdleMinSetTm1 : Constant  Value=CcBSP_DCChrgPosTempHiThrd_C
  KeMDPR_t_EngChrgBatIdleMinSetTm10 : Constant  Value=CcBSP_DCChrgNegTempHiThrd_C
  LDP_GeLDP_CC2St_enum : AIWAYS_Powertrain_BMS_lib/Signals/OverWrite  OverWrite_Value=CbBSP_DCChrgNegTempSafOvr_flg  OverWrite_flag=CbBSP_DCChrgNegTempSafOvrSwt_flg
  LDP_GeLDP_CC2St_enum1 : AIWAYS_Powertrain_BMS_lib/Signals/OverWrite  OverWrite_Value=CbBSP_DCChrgPosTempSafOvr_flg  OverWrite_flag=CbBSP_DCChrgPosTempSafOvrSwt_flg
  Logical1 : Logic  Inputs=4  OutDataTypeStr=boolean
  Logical2 : Logic  Inputs=4  OutDataTypeStr=boolean
  Relational Operator{1..4} (4 alike) : RelationalOperator  Operator===  OutDataTypeStr=boolean
  Terminator : Terminator
  Terminator1 : Terminator
  GbBSP_DCChrgNegTempSaf_flg : Outport
  GbBSP_DCChrgPosTempSaf_flg : Outport  Port=2
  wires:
  Comparison1/1 -> Logical1/4
  Relational Operator3/1 -> Logical1/2
  GcLDP_ChrgTempNeg_C/1 -> Bus Creator/4
  GbLDP_DCChrgNegTempSTGFlt_flg/1 -> Bus Creator/3
  GbLDP_DCChrgNegTempSTVFlt_flg/1 -> Bus Creator/2
  KeMDPR_t_EngChrgBatIdleMinSetTm10/1 -> Comparison1/2
  Constant1/1 -> Relational Operator1/2
  Relational Operator1/1 -> Logical1/3
  Constant3/1 -> Comparison2/1
  Comparison2/1 -> Terminator/1
  Data Type Conversion/1 -> Comparison2/2
  GeCTC_CtrCtlConnMode_enum/1 -> Bus Creator/1
  Constant4/1 -> Relational Operator3/2
  Logical1/1 -> LDP_GeLDP_CC2St_enum/1
  LDP_GeLDP_CC2St_enum/1 -> GbBSP_DCChrgNegTempSaf_flg/1  "GbBSP_DCChrgNegTempSaf_flg"
  LDP_GeLDP_CC2St_enum1/1 -> GbBSP_DCChrgPosTempSaf_flg/1  "GbBSP_DCChrgPosTempSaf_flg"
  Data Type Conversion1/1 -> Comparison4/2
  Constant6/1 -> Relational Operator4/2
  Relational Operator4/1 -> Logical2/2
  Relational Operator2/1 -> Logical2/3
  GbLDP_DCChrgPosTempSTVFlt_flg/1 -> Bus Creator/5
  GcLDP_ChrgTempPos_C/1 -> Bus Creator/7
  Constant5/1 -> Comparison4/1
  Comparison4/1 -> Terminator1/1
  KeMDPR_t_EngChrgBatIdleMinSetTm1/1 -> Comparison3/2
  GbLDP_DCChrgPosTempSTGFlt_flg/1 -> Bus Creator/6
  Comparison3/1 -> Logical2/4
  Constant2/1 -> Relational Operator2/2
  Logical2/1 -> LDP_GeLDP_CC2St_enum1/1
  Bus Creator/1 -> Bus Selector3/1, Bus Selector1/1, Bus Selector2/1, Bus Selector/1
  Bus Selector/1 -> Data Type Conversion/1  "<GeCTC_CtrCtlConnMode_enum>"
  Bus Selector/2 -> Relational Operator3/1  "<GbLDP_DCChrgNegTempSTVFlt_flg>"
  Bus Selector/3 -> Relational Operator1/1  "<GbLDP_DCChrgNegTempSTGFlt_flg>"
  Bus Selector/4 -> Comparison1/1  "<GcLDP_ChrgTempNeg_C>"
  Bus Selector1/1 -> Data Type Conversion1/1  "<GeCTC_CtrCtlConnMode_enum>"
  Bus Selector1/2 -> Relational Operator4/1  "<GbLDP_DCChrgPosTempSTVFlt_flg>"
  Bus Selector1/3 -> Relational Operator2/1  "<GbLDP_DCChrgPosTempSTGFlt_flg>"
  Bus Selector1/4 -> Comparison3/1  "<GcLDP_ChrgTempPos_C>"
  Data Type Conversion3/1 -> Comparison5/1
  Constant7/1 -> Comparison5/2
  GeLDP_CC2St_enum/1 -> Bus Creator/8
  Bus Selector2/1 -> Data Type Conversion3/1  "<GeLDP_CC2St_enum>"
  Comparison5/1 -> Logical1/1
  Comparison6/1 -> Logical2/1
  Bus Selector3/1 -> Data Type Conversion2/1  "<GeLDP_CC2St_enum>"
  Constant8/1 -> Comparison6/2
  Data Type Conversion2/1 -> Comparison6/1

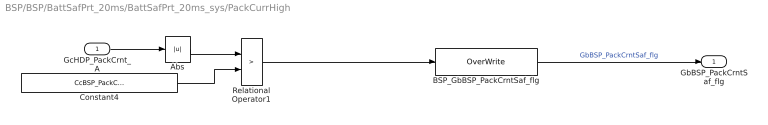
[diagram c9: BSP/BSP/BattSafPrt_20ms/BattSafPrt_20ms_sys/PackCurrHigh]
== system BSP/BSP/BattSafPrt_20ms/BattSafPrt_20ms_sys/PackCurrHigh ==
  GcHDP_PackCrnt_A : Inport
  Abs : Abs
  BSP_GbBSP_PackCrntSaf_flg : AIWAYS_Powertrain_BMS_lib/Signals/OverWrite  OverWrite_Value=CbBSP_PackCrntSafOvr_flg  OverWrite_flag=CbBSP_PackCrntSafOvrSwt_flg
  Constant4 : Constant  Value=CcBSP_PackCurrSaf_A
  Relational Operator1 : RelationalOperator  Operator=>  OutDataTypeStr=boolean
  GbBSP_PackCrntSaf_flg : Outport
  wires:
  Relational Operator1/1 -> BSP_GbBSP_PackCrntSaf_flg/1
  BSP_GbBSP_PackCrntSaf_flg/1 -> GbBSP_PackCrntSaf_flg/1  "GbBSP_PackCrntSaf_flg"
  Constant4/1 -> Relational Operator1/2
  GcHDP_PackCrnt_A/1 -> Abs/1
  Abs/1 -> Relational Operator1/1
